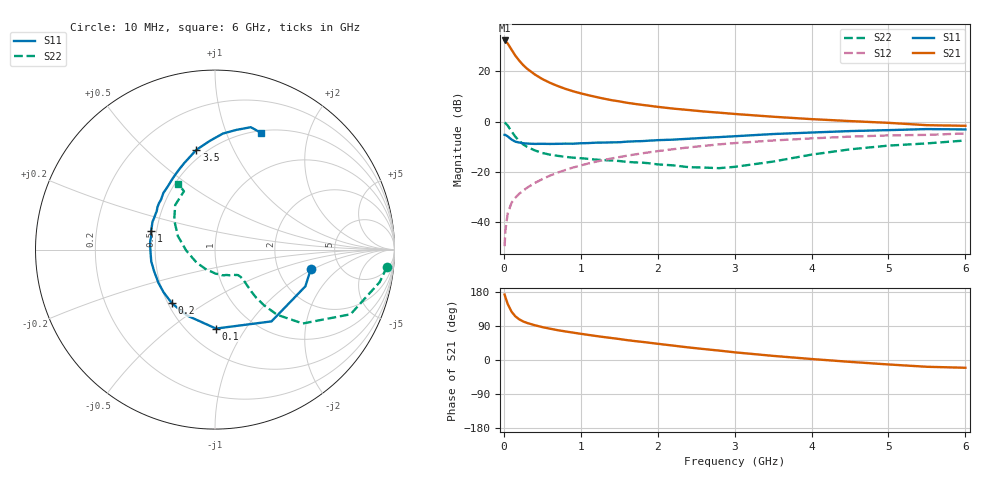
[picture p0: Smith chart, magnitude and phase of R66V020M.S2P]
! SIEMENS Small Signal Semiconductors
! BFR193
! Si NPN RF Bipolar Junction Transistor in SOT23
! VCE = 6 V  IC = 20 mA
! Common Emitter S-Parameters:  May  1996
# GHz  S  MA  R  50
!  f  S11  S21  S12  S22
! GHz  MAG  ANG  MAG  ANG  MAG  ANG  MAG  ANG
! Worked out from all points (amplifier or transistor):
!   36 points, 10 MHz to 6 GHz, reference 50 ohm
!   highest |S21| = 32.3 dB at 10 MHz (marker M1)
!   |S21| within 3 dB of that: start of sweep to 86.5 MHz
!   unconditionally stable (mu >= 1): 582.5 MHz to 1.976 GHz
!   at 250 MHz: K = 0.82, MSG = 25.1 dB, |S12| = -27.5 dB
!   at 1.4 GHz: K = 1.03, MAG = 10.6 dB, |S12| = -14.7 dB
!   at 6 GHz: K = 0.94, MSG = 1.5 dB, |S12| = -4.7 dB
!   lowest NFmin = 1.40 dB at 450 MHz
!   S11 on the Smith chart (normalised r, x): 10 MHz: 3.08, -0.94; 100 MHz: 0.68, -0.74; 200 MHz: 0.52, -0.37; 1 GHz: 0.47, +0.11; 3.5 GHz: 0.45, +0.73; 6 GHz: 0.52, +1.33
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0.01  0.5449 -11.3  41.45 172.7  0.0033 84.3  0.9633 -5.7
0.02  0.5436 -22.1  40.37 165.8  0.0067 85.5  0.9349 -11.2
0.05  0.509 -51.8  36.06 148.0  0.0148 72.9  0.8368 -25.5
0.1  0.44 -89.3  27.18 127.6  0.0242 63.7  0.6392 -40.1
0.15  0.3989 -113.1  20.61 115.1  0.0305 61.8  0.501 -46.4
0.2  0.3836 -128.7  16.41 107.3  0.0366 62.7  0.4135 -48.6
0.25  0.3722 -140.4  13.46 101.8  0.042 64.2  0.3534 -49.4
0.3  0.3658 -149.4  11.41 97.9  0.0479 65.1  0.3153 -49.2
0.4  0.36 -160.8  8.765 91.9  0.0597 66.7  0.2682 -48.1
0.5  0.3613 -169.5  7.058 86.8  0.0715 68.1  0.2372 -47.0
0.6  0.3593 -176.7  5.937 82.6  0.084 68.6  0.2199 -46.7
0.7  0.3611 177.5  5.124 78.7  0.0966 68.7  0.2083 -46.8
0.8  0.3642 172.8  4.504 75.4  0.1087 67.9  0.1987 -47.3
1  0.3709 163.7  3.659 69.2  0.1339 66.9  0.1867 -49.2
1.1  0.3739 160.6  3.358 66.2  0.1469 66.1  0.1811 -51.4
1.3  0.3825 152.2  2.87 60.6  0.1722 64.1  0.1708 -55.2
1.6  0.3991 143.3  2.377 52.5  0.2092 60.7  0.1581 -63.8
2.2  0.4378 127.3  1.819 38.0  0.2823 53.0  0.1346 -88.0
3.5  0.566 100.5  1.252 10.9  0.421 33.7  0.1599 -177.8
4.5  0.6482 86.1  1.026 -4.9  0.5023 19.5  0.2805 144.1
5.5  0.7105 73.7  0.85 -17.9  0.5447 5.2  0.3684 118.0
6  0.6991 68.4  0.826 -20.5  0.5816 1.1  0.4212 119.3
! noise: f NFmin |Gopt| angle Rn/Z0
0.45  1.4  0.3  160  0.1
0.9  1.45  0.34  172  0.11
1.8  2.2  0.56  -148  0.2
